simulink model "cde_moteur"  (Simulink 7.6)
settings: Solver=ode15s  StartTime=0.0  StopTime=10  FixedStep=0.1  RelTol=1e-3
StopFcn:
  | close all, clc
  | load cde_moteur.mat
  | plotyy(x(1,:),x(2,:),x(1,:),x(3,:))
  | title('Position et vitesse angulaires de l''arbre du moteur')
  | xlabel('temps')
  | grid
libraries: fl_lib x9, elec_lib x5, nesl_utility x5

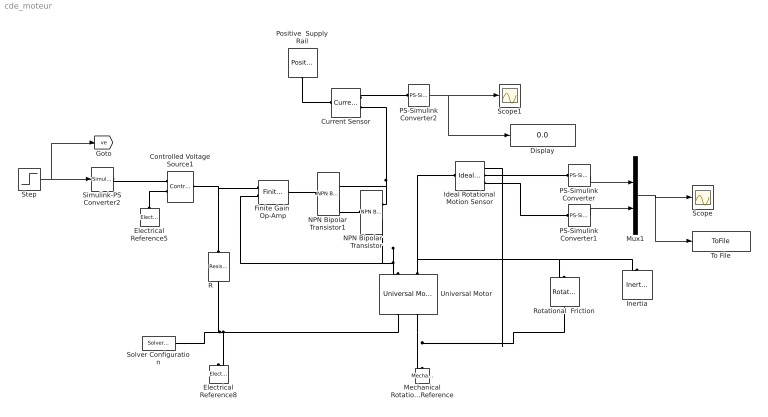
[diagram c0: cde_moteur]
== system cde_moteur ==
  Controlled Voltage Source1 : fl_lib/Electrical/Electrical Sources/Controlled Voltage Source  DialogController=NetworkEngine.DynNeDlgSource  SystemSampleTime=-1  i_Log=off  v_Log=off  LocalVarNames=|current|voltage|power  LocalVarDescs=|Current (A)|Voltage (V)|Power (W)  LocalVarLogging=[0 0 0]
  Current Sensor : fl_lib/Electrical/Electrical Sensors/Current Sensor  DialogController=NetworkEngine.DynNeDlgSource  SystemSampleTime=-1  i1_Log=off  v1_Log=off  LocalVarNames=|i1|v1  LocalVarDescs=|i1|v1  LocalVarLogging=[0 0]
  Display : Display
  Electrical Reference5 : fl_lib/Electrical/Electrical Elements/Electrical Reference  DialogController=NetworkEngine.DynNeDlgSource  SystemSampleTime=-1  i_Log=off  LocalVarNames=|i  LocalVarDescs=|i  LocalVarLogging=[]
  Electrical Reference8 : fl_lib/Electrical/Electrical Elements/Electrical Reference  DialogController=NetworkEngine.DynNeDlgSource  SystemSampleTime=-1  i_Log=off  LocalVarNames=|i  LocalVarDescs=|i  LocalVarLogging=[]
  Finite Gain  Op-Amp : elec_lib/Integrated Circuits/Finite Gain Op-Amp  DialogController=NetworkEngine.DynNeDlgSource  SystemSampleTime=-1  A=1000  Rin=1e+06 Ohm  Rout=100 Ohm  Vmin=-15 V  Vmax=15 V  LocalVarNames=|power  LocalVarDescs=|Dissipated power (W)  LocalVarLogging=0
  Ideal Rotational Motion Sensor : fl_lib/Mechanical/Mechanical Sensors/Ideal Rotational Motion Sensor  DialogController=NetworkEngine.DynNeDlgSource  SystemSampleTime=-1  offset=0 rad  w_Log=off  t_Log=off  phi_Log=off  LocalVarNames=|w|t|phi  LocalVarDescs=|w|t|phi  LocalVarLogging=[0 0 0]
  Inertia : fl_lib/Mechanical/Rotational Elements/Inertia  DialogController=NetworkEngine.DynNeDlgSource  SystemSampleTime=-1  inertia=5 kg*m^2  initial_velocity=0 rad/s  t_Log=off  LocalVarNames=|t  LocalVarDescs=|t  LocalVarLogging=0
  Mechanical Rotational Reference : fl_lib/Mechanical/Rotational Elements/Mechanical Rotational Reference  DialogController=NetworkEngine.DynNeDlgSource  SystemSampleTime=-1  t_Log=off  LocalVarNames=|t  LocalVarDescs=|t  LocalVarLogging=0
  Mux1 : Mux  Inputs=2
  NPN Bipolar Transistor : elec_lib/Semiconductor Devices/NPN Bipolar Transistor  DialogController=NetworkEngine.DynNeDlgSource  SystemSampleTime=-1  parameterization=1  BF=100  IS=1e-14 A  VAF=200 V  hfe=100  hoe=5e-5 1/Ohm  Ic_h=1 mA  V1=0.55 V  I1=0.5 mA  BR=1  Tmeas=25 C  RC=0.01 Ohm  RE=1e-4 Ohm  RB=1 Ohm  C_BC=5 pF  C_BE=5 pF  TF=0 us  TR=0 us  LocalVarLogging=[]
  NPN Bipolar Transistor1 : elec_lib/Semiconductor Devices/NPN Bipolar Transistor  DialogController=NetworkEngine.DynNeDlgSource  SystemSampleTime=-1  parameterization=1  BF=100  IS=1e-14 A  VAF=200 V  hfe=100  hoe=5e-5 1/Ohm  Ic_h=1 mA  V1=0.55 V  I1=0.5 mA  BR=1  Tmeas=25 C  RC=0.01 Ohm  RE=1e-4 Ohm  RB=1 Ohm  C_BC=5 pF  C_BE=5 pF  TF=0 us  TR=0 us  LocalVarLogging=[]
  PS-Simulink Converter : nesl_utility/PS-Simulink Converter  DialogController=NetworkEngine.DynNeUtilDlgSource  SystemSampleTime=-1  PhysicalDomain=network_engine_domain  LeftPortType=input  RightPortType=output  SubClassName=ps_output  Unit=1  AffineConversion=off
  PS-Simulink Converter1 : nesl_utility/PS-Simulink Converter  DialogController=NetworkEngine.DynNeUtilDlgSource  SystemSampleTime=-1  PhysicalDomain=network_engine_domain  LeftPortType=input  RightPortType=output  SubClassName=ps_output  Unit=1  AffineConversion=off
  PS-Simulink Converter2 : nesl_utility/PS-Simulink Converter  DialogController=NetworkEngine.DynNeUtilDlgSource  SystemSampleTime=-1  PhysicalDomain=network_engine_domain  LeftPortType=input  RightPortType=output  SubClassName=ps_output  Unit=A  AffineConversion=off
  Positive  Supply Rail : elec_lib/Sources/Positive Supply Rail  DialogController=NetworkEngine.DynNeDlgSource  SystemSampleTime=-1  v0=50 V  current_Log=off  voltage_Log=off  power_Log=off  LocalVarNames=|current|voltage|power  LocalVarDescs=|Current (A)|Voltage (V)|Power (W)  LocalVarLogging=[0 0 0]
  R : fl_lib/Electrical/Electrical Elements/Resistor  DialogController=NetworkEngine.DynNeDlgSource  SystemSampleTime=-1  R=1 MOhm  i_Log=off  v_Log=off  LocalVarNames=|current|voltage|power  LocalVarDescs=|Resistor current (A)|Voltage across resistor (V)|Power (W)  LocalVarLogging=[0 0 0]
  Rotational  Friction : fl_lib/Mechanical/Rotational Elements/Rotational Friction  DialogController=NetworkEngine.DynNeDlgSource  SystemSampleTime=-1  brkwy_trq=1e-6 N*m  Col_trq=1e-6 N*m  visc_coef=5 N*m/(rad/s)  trans_coef=10 s/rad  vel_thr=1e-4 rad/s  t_Log=off  w_Log=off  LocalVarNames=|t|w  LocalVarDescs=|t|w  LocalVarLogging=[0 0]
  Scope : Scope
  Scope1 : Scope
  Simulink-PS Converter2 : nesl_utility/Simulink-PS Converter  DialogController=NetworkEngine.DynNeUtilDlgSource  SystemSampleTime=-1  PhysicalDomain=network_engine_domain  LeftPortType=input  RightPortType=output  SubClassName=ps_input  Unit=1  AffineConversion=off  InputFilterTimeConstant=.001  UdotUserProvided=0
  Solver Configuration : nesl_utility/Solver Configuration  DialogController=NetworkEngine.DynNeUtilDlgSource  SystemSampleTime=-1  PhysicalDomain=network_engine_domain  LeftPortType=input  RightPortType=generic  SubClassName=solver  Accelerate=off  Profile=off  ResidualTolerance=1e-40  MaxNonlinIter=12  MaxModeIter=2  DoFixedCost=off  UseLocalSampling=off  DoDC=on  LinearAlgebra=Full  LocalSolverSampleTime=.001  LocalSolverChoice=NE_BACKWARD_EULER_ADVANCER  UseLocalSolver=off
  Step : Step  After=24  SampleTime=0
  To File : ToFile  Filename=cde_moteur  MatrixName=x
  Universal Motor : elec_lib/Actuators & Drivers/Rotational Actuators/Universal Motor  DialogController=NetworkEngine.DynNeDlgSource  SystemSampleTime=-1  parameterization=3  Ra=132.8 Ohm  Laf=0.1722 s*V/rad/A  w_rated=6.5e+3 rpm  P_rated=75 W  V_dc=50 V  T_max=0.39 N*m  P_in=160 W  V_ac=240 V  I_ac=0.8 A  w_ac=50 Hz  Ltot=0.525 H  J=2e-4 kg*m^2  lam=1e-6 N*m/(rad/s)  speed0=0 rpm  current_Log=off  voltage_Log=off  power_Log=off  i2r_Log=off  torque_Log=off  speed_Log=off  LocalVarNames=|current|voltage|power|i2r|torque|speed  LocalVarDescs=|Current (A)|Voltage (V)|Power (W)|Electrical losses (W)|Torque (Nm)|Angular speed (rad/s)  LocalVarLogging=[0 0 0 0 0 0]
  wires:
  Mux1/1 -> To File/1, Scope/1
  Step/1 -> Simulink-PS Converter2/1, [ve]
  PS-Simulink Converter1/1 -> Mux1/2
  PS-Simulink Converter/1 -> Mux1/1
  PS-Simulink Converter2/1 -> Display/1, Scope1/1
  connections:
  Simulink-PS Converter2/RConn1 -- Controlled Voltage Source1/RConn1
  Electrical Reference5/LConn1 -- Controlled Voltage Source1/RConn2
  R/LConn1 -- Finite Gain  Op-Amp/LConn1 -- Controlled Voltage Source1/LConn1
  Universal Motor/LConn1 -- NPN Bipolar Transistor/RConn2 -- Finite Gain  Op-Amp/LConn2
  Universal Motor/RConn2 -- Mechanical Rotational Reference/LConn1 -- Rotational  Friction/RConn1 -- Ideal Rotational Motion Sensor/RConn1
  Ideal Rotational Motion Sensor/RConn2 -- PS-Simulink Converter/LConn1
  Universal Motor/LConn2 -- Ideal Rotational Motion Sensor/LConn1 -- Rotational  Friction/LConn1 -- Inertia/LConn1
  Ideal Rotational Motion Sensor/RConn3 -- PS-Simulink Converter1/LConn1
  Current Sensor/RConn2 -- NPN Bipolar Transistor/RConn1 -- NPN Bipolar Transistor1/RConn1
  Positive  Supply Rail/RConn1 -- Current Sensor/LConn1
  Current Sensor/RConn1 -- PS-Simulink Converter2/LConn1
  Universal Motor/RConn1 -- Electrical Reference8/LConn1 -- R/RConn1 -- Solver Configuration/RConn1
  NPN Bipolar Transistor1/LConn1 -- Finite Gain  Op-Amp/RConn1
  NPN Bipolar Transistor1/RConn2 -- NPN Bipolar Transistor/LConn1
